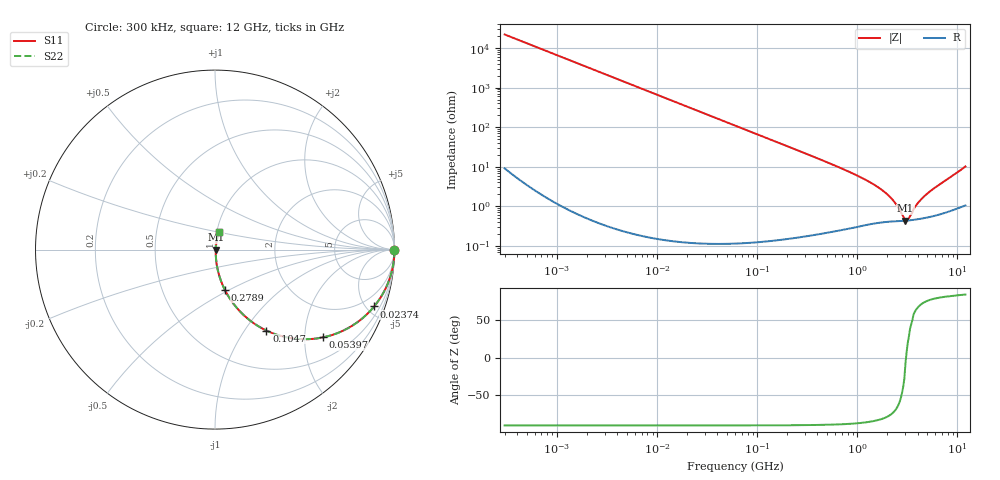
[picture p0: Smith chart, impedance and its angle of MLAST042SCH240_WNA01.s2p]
! MLAST042SCH240_WNA01  S-PARAMETER MODEL  ( General Type )
! Model Generated by TAIYO YUDEN Corporation (http://www.ty-top.com)
! Version 1.0
! TAIYO YUDEN Control No. 150820
! Copyright(c) 2015 TAIYO YUDEN CO.,LTD. All Rights Reserved.
! Product Description (link to TY-COMPAS)
! https://ds.yuden.co.jp/TYCOMPAS/or/detail?pn=MLAST042SCH240JWNA01&u=M
! Products Name : Multilayer Ceramic Capacitors
! Characteristics :
!  Capacitance : 24 pF , Rated Voltage : 25V , TCC : CH / C0H
!  Case Size : 0.4 x 0.2 / 0.016 x 0.008 [mm/inch] , Thickness : 0.2 / 0.008 [mm/inch]
!  (Conditions: Temperature = 25 degC , DC Bias Current/Voltage = 0A / 0V)
! External Node Assignments :
!  1  o---| |---o  2
! GND o---------o GND
! Frequency Range : 0.3MHz  -  12000MHz  [ 401 STEP ]
# MHz S RI R 50
! Freq[MHz].  S11 Real  S11 Imag  S21 Real  S21 Imag  S12 Real  S12 Imag  S22 Real  S22 Imag
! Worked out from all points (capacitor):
!   401 points, 300 kHz to 12 GHz, reference 50 ohm
!   read as one part in series: C = 24 pF near 316.3 kHz
!   lowest |Z| = 432 mohm at 3.026 GHz (marker M1)
!   series resonance near 3.065 GHz, so ESL is about 110 pH
!   S11 on the Smith chart (normalised r, x): 300 kHz: open; 23.74 MHz: 1.00, -5.59; 53.97 MHz: 1.00, -2.46; 104.7 MHz: 1.00, -1.27; 278.9 MHz: 1.00, -0.47; 12 GHz: 1.02, +0.20
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0.3  1 -0.00452  2.23e-05 0.00452  2.23e-05 0.00452  1 -0.00452
1.769972  0.9993 -0.0266  0.000714 0.0266  0.000714 0.0266  0.9993 -0.0266
4.84353  0.9947 -0.0726  0.00531 0.0726  0.00531 0.0726  0.9947 -0.0726
10.44266  0.9758 -0.1535  0.0242 0.1535  0.0242 0.1535  0.9758 -0.1535
23.73947  0.8865 -0.317  0.1135 0.317  0.1135 0.317  0.8865 -0.317
35.32224  0.7792 -0.4145  0.2208 0.4145  0.2208 0.4145  0.7792 -0.4145
53.9673  0.6018 -0.4891  0.3982 0.4891  0.3982 0.4891  0.6018 -0.4891
60  0.5501 -0.497  0.4499 0.497  0.4499 0.497  0.5501 -0.497
104.6549  0.2868 -0.4513  0.7132 0.4513  0.7132 0.4513  0.2868 -0.4513
164.1901  0.1407 -0.346  0.8593 0.346  0.8593 0.346  0.1407 -0.346
278.9009  0.0542 -0.2229  0.9458 0.2229  0.9458 0.2229  0.0542 -0.2229
353.9943  0.0348 -0.1783  0.9652 0.1783  0.9652 0.1783  0.0348 -0.1783
1166.079  0.00563 -0.0485  0.9944 0.0485  0.9944 0.0485  0.00563 -0.0485
1645.489  0.00464 -0.0288  0.9954 0.0288  0.9954 0.0288  0.00464 -0.0288
2088.533  0.00437 -0.0173  0.9956 0.0173  0.9956 0.0173  0.00437 -0.0173
2448.343  0.00428 -0.0102  0.9957 0.0102  0.9957 0.0102  0.00428 -0.0102
2870.14  0.00425 -0.00337  0.9957 0.00337  0.9957 0.00337  0.00425 -0.00337
3026.31  0.00427 -0.000532  0.9957 0.000532  0.9957 0.000532  0.00427 -0.000532
3276.641  0.00437 0.00238  0.9956 -0.00238  0.9956 -0.00238  0.00437 0.00238
3944.255  0.00475 0.0102  0.9952 -0.0102  0.9952 -0.0102  0.00475 0.0102
4875.354  0.00547 0.019  0.9945 -0.019  0.9945 -0.019  0.00547 0.019
12000  0.0202 0.0978  0.9798 -0.0978  0.9798 -0.0978  0.0202 0.0978
